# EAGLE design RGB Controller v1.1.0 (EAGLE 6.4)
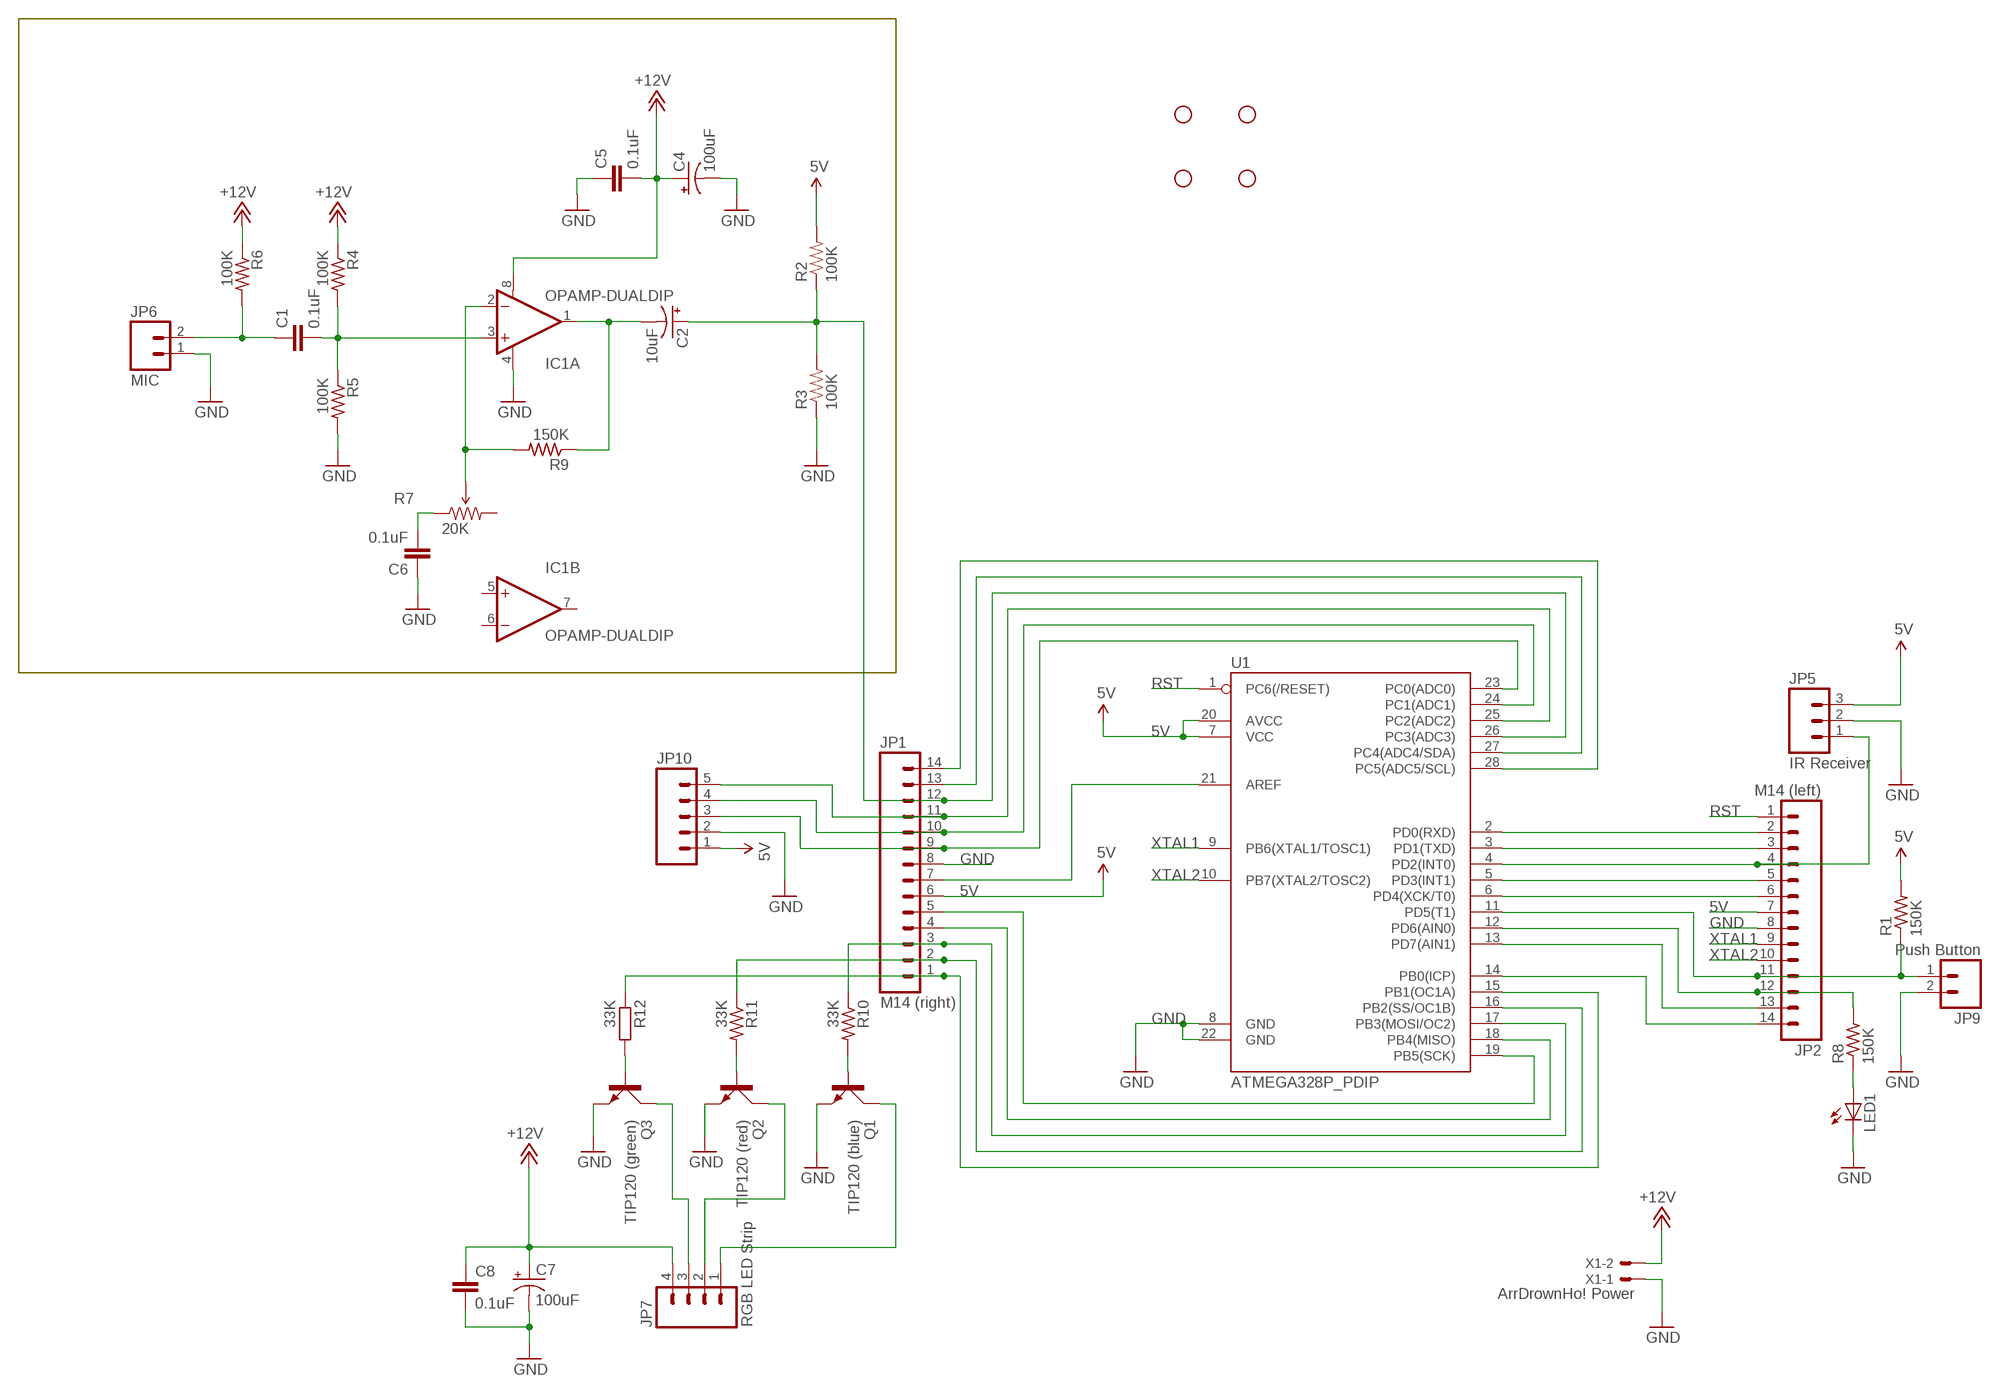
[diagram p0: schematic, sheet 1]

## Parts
C1  0.1uF  CAPPTH  [CAP-PTH-SMALL]
C2  10uF  CAP_POLPTH2  [CPOL-RADIAL-10UF-25V]
C4  100uF  CAP_POLPTH1  [CPOL-RADIAL-100UF-25V]
C5  0.1uF  CAPPTH  [CAP-PTH-SMALL]
C6  0.1uF  CAPPTH  [CAP-PTH-SMALL]
C7  100uF  CAP_POLPTH1  [CPOL-RADIAL-100UF-25V]
C8  0.1uF  CAPPTH  [CAP-PTH-SMALL]
IC1  OPAMP-DUALDIP  [DIP08]
JP1  M14 (right)  M14  [1X14]
JP2  M14 (left)  M14  [1X14]
JP5  IR Receiver  M03PTH  [1X03]
JP6  MIC  M02PTH  [1X02]
JP7  RGB LED Strip  M04PTH  [1X04]
JP9  Push Button  M02PTH  [1X02]
JP10  M05PTH  [1X05]
LED1  LED3MM  [LED3MM]
Q1  TIP120 (blue)  TIP41C  [TO220AV]
Q2  TIP120 (red)  TIP41C  [TO220AV]
Q3  TIP120 (green)  TIP41C  [TO220AV]
R1  150K  R-US_0207/2V  [0207/2V]
R2  100K  RESISTORAXIAL-0.3  [AXIAL-0.3]
R3  100K  RESISTORAXIAL-0.3  [AXIAL-0.3]
R4  100K  R-US_0207/2V  [0207/2V]
R5  100K  R-US_0207/2V  [0207/2V]
R6  100K  R-US_0207/2V  [0207/2V]
R7  20K  TRIMPOTPTH  [TRIM_POT_PTH]
R8  150K  R-US_0207/2V  [0207/2V]
R9  150K  R-US_0207/2V  [0207/2V]
R10  33K  R-US_0207/2V  [0207/2V]
R11  33K  R-US_0207/2V  [0207/2V]
R12  33K  R-EU_0411/3V  [0411V]
STANDOFF1  STAND-OFF  [STAND-OFF]
STANDOFF2  STAND-OFF  [STAND-OFF]
STANDOFF3  STAND-OFF  [STAND-OFF]
STANDOFF4  STAND-OFF  [STAND-OFF]
U1  ATMEGA328P_PDIP  [DIL28-3]
X1  ArrDrownHo! Power  C-GRID-02-70543  [70543-02]

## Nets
5V: JP1.6 JP2.7 JP5.3 JP10.1 R1.2 R2.P$2 U1.7(VCC) U1.20(AVCC)
+12V: C4.1(+) C5.2 C7.1(+) C8.1 IC1.8(A:V+) JP7.4 R4.1 R6.1 X1.2
AREF: JP1.7 U1.21(AREF)
GND: C4.2(-) C5.1 C6.1 C7.2(-) C8.2 IC1.4(A:V-) JP1.8 JP2.8 JP5.2 JP6.1 JP9.2 JP10.2 LED1.K(C) Q1.E Q2.E Q3.E R3.P$1 R5.2 U1.8(GND) U1.22(GND) X1.1
N$1: JP2.2 U1.2(PD0(RXD))
N$2: JP2.3 U1.3(PD1(TXD))
N$3: JP2.4 JP5.1 U1.4(PD2(INT0))
N$4: JP2.5 U1.5(PD3(INT1))
N$5: JP2.6 U1.6(PD4(XCK/T0))
N$6: LED1.A R8.1
N$7: JP2.12 R8.2 U1.12(PD6(AIN0))
N$8: JP2.13 U1.13(PD7(AIN1))
N$9: JP1.9 JP10.3 U1.23(PC0(ADC0))
N$10: JP1.10 JP10.4 U1.24(PC1(ADC1))
N$11: JP1.11 JP10.5 U1.25(PC2(ADC2))
N$12: JP7.2 Q2.C
N$13: JP1.13 U1.27(PC4(ADC4/SDA))
N$14: JP1.14 U1.28(PC5(ADC5/SCL))
N$15: JP1.1 R12.1 U1.15(PB1(OC1A))
N$16: JP2.14 U1.14(PB0(ICP))
N$17: JP1.5 U1.19(PB5(SCK))
N$18: JP1.4 U1.18(PB4(MISO))
N$19: JP1.3 R10.1 U1.17(PB3(MOSI/OC2))
N$20: JP1.2 R11.1 U1.16(PB2(SS/OC1B))
N$21: C2.1(+) JP1.12 R2.P$1 R3.P$2 U1.26(PC3(ADC3))
N$22: C2.2(-) IC1.1(A:OUT) R9.1
N$25: IC1.2(A:-IN) R7.2(WIPER) R9.2
N$26: Q2.B R11.2
N$27: C1.2 IC1.3(A:+IN) R4.2 R5.1
N$28: C1.1 JP6.2 R6.2
N$29: C6.2 R7.1(CCW)
N$30: Q3.B R12.2
N$31: Q1.B R10.2
N$33: JP7.3 Q3.C
N$35: JP7.1 Q1.C
N$37: JP2.11 JP9.1 R1.1 U1.11(PD5(T1))
RST: JP2.1 U1.1(PC6(/RESET))
XTAL1: JP2.9 U1.9(PB6(XTAL1/TOSC1))
XTAL2: JP2.10 U1.10(PB7(XTAL2/TOSC2))
Unconnected: IC1.5(B:+IN) IC1.6(B:-IN) IC1.7(B:OUT) R7.3(CW)

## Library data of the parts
C1 C5 C6 C8 = SparkFun-Capacitors:CAP: Capacitor
C2 C4 C7 = SparkFun-Capacitors:CAP_POL: Capacitor Polarized
IC1 = SparkFun-AnalogIC:OPAMP-DUAL: Generic op-amp footprint
JP1 JP2 = SparkFun-Connectors:M14: Header 14 Standard 14-pin 0.1" header. Use with straight break away headers (SKU : PRT-00116), right angle break away headers (PRT-00553), swiss pins (PRT-00743), machine pins (PRT-00117), and female headers (PRT-00115).
JP5 = SparkFun-Connectors:M03: Header 3 Standard 3-pin 0.1" header. Use with straight break away headers (SKU : PRT-00116), right angle break away headers (PRT-00553), swiss pins (PRT-00743), machine pins (PRT-00117), and female headers (PRT-00115). Molex polarized connector foot print use with SKU : PRT-08232 with associated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
JP6 JP9 = SparkFun-Connectors:M02: Header 2
JP7 = SparkFun-Connectors:M04: Header 4 Standard 4-pin 0.1" header. Use with straight break away headers (SKU : PRT-00116), right angle break away headers (PRT-00553), swiss pins (PRT-00743), machine pins (PRT-00117), and female headers (PRT-00115). Molex polarized connector foot print use with SKU : PRT-08231 with associated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
JP10 = SparkFun-Connectors:M05: Header 5 Standard 5-pin 0.1" header. Use with straight break away headers (SKU : PRT-00116), right angle break away headers (PRT-00553), swiss pins (PRT-00743), machine pins (PRT-00117), and female headers (PRT-00115). Molex polarized connector foot print use with SKU : PRT-08230 with associated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
LED1 = SparkFun-LED:LED: LEDs
Q1-Q3 = transistor-power:TIP41C: NPN TRANSISTOR
R1 R4-R6 R8-R11 = resistor:R-US_: RESISTOR, American symbol
R2 R3 = SparkFun-Passives:RESISTOR: Resistor
R7 = SparkFun-Electromechanical:TRIMPOT: Various small potentiometers for "set-and-forget" applications
R12 = resistor:R-EU_: RESISTOR, European symbol
STANDOFF1-STANDOFF4 = SparkFun-Electromechanical:STAND-OFF: #4 Stand Off
U1 = SparkFun-DigitalIC:ATMEGA328P_PDIP: uC used in the Arduino 32kb flash, 1k EEPROM, 2k SRAM This is the through-hole version of this chip.
X1 = con-molex:C-GRID-02: CONNECTOR; OC_FARNELL: unknown; OC_NEWARK: unknown

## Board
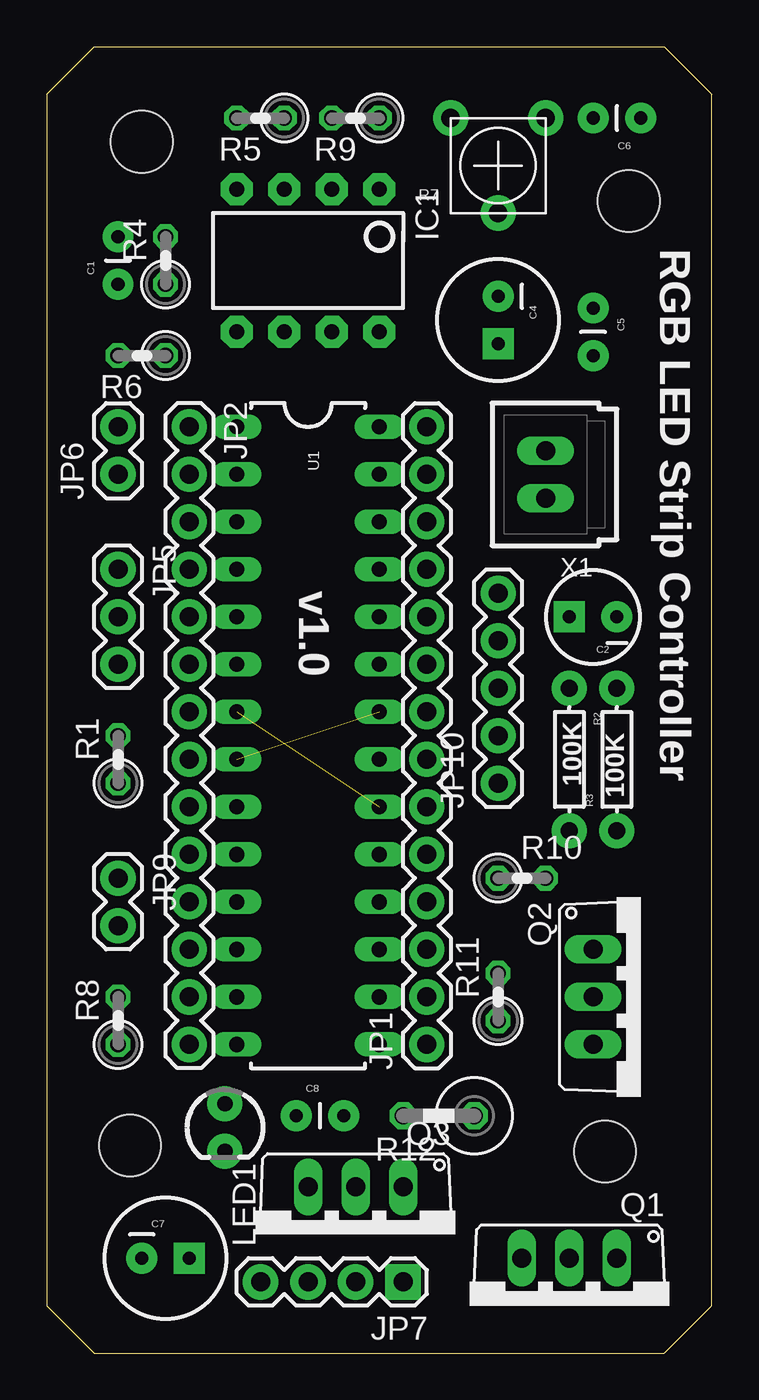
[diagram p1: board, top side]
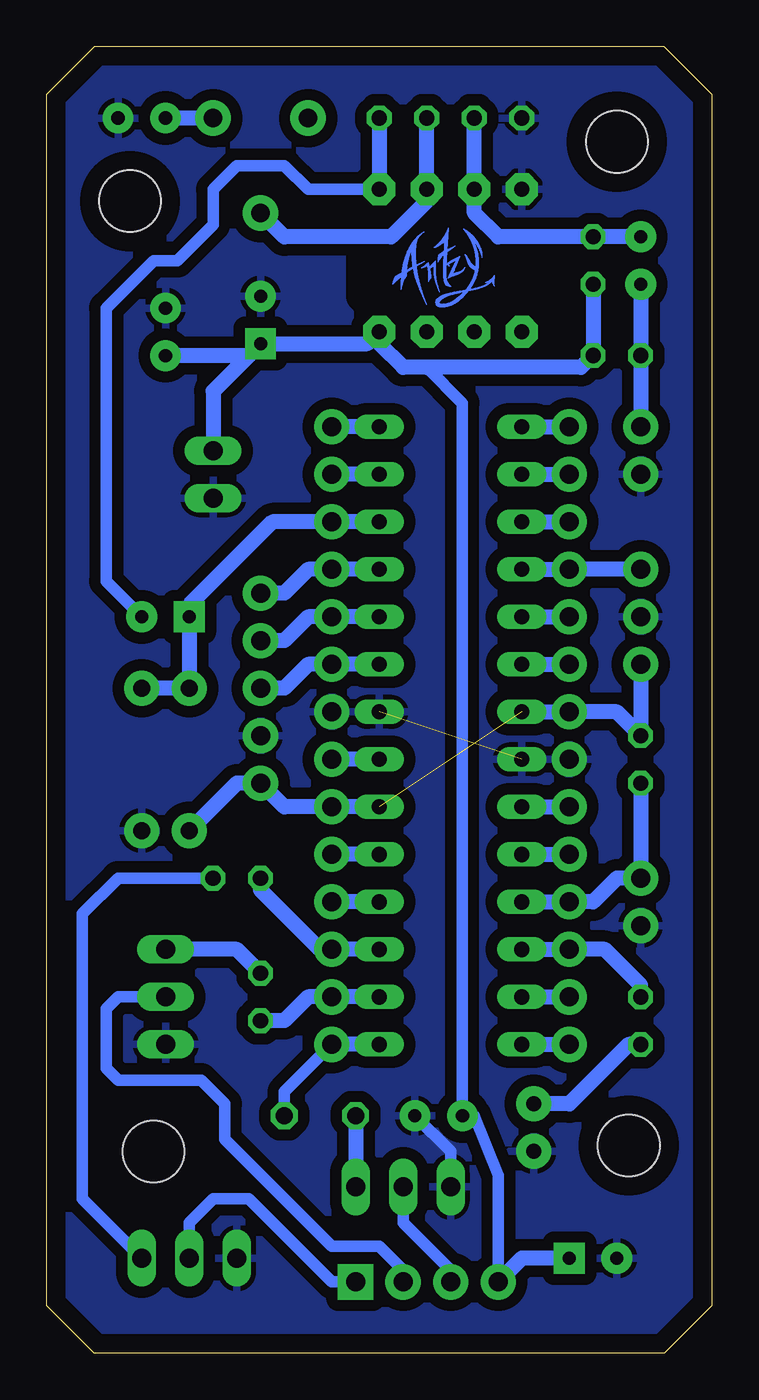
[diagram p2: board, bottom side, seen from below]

Size 35.56 x 69.85 mm. Coordinates in mm from the lower left corner, seen from the top.
Outline: 35.56,2.54 35.56,67.31 33.02,69.85 2.54,69.85 0,67.31 0,2.54 2.54,0 33.02,0 35.56,2.54
Copper layers (1*16): Top 0.035mm / dielectric 1.5mm / Bottom 0.035mm
Design rules "default *": minimum track width 10mil, minimum drill 24mil, track to track 8mil, track to pad 8mil, pad to pad 8mil, via to via 8mil, smd to smd 8mil, copper to edge 40mil, drill to drill 8mil, minimum pad ring 10mil, minimum via ring 8mil, stop-mask expansion 4mil, vias tented up to drill 0mil, thermal gap 10mil
bRestrict: area 17.5,56.1 to 18.9,58.7

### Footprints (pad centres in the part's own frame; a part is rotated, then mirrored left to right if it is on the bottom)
CAP-PTH-SMALL = drill 0.7 pad 1.651: 1 0,0; 2 2.54,0
CPOL-RADIAL-10UF-25V = drill 0.7 pad 1.651 square: 1 1.27,0 | drill 0.7 pad 1.651: 2 -1.27,0
CPOL-RADIAL-100UF-25V = drill 0.7 pad 1.651 square: 1 1.27,0 | drill 0.7 pad 1.651: 2 -1.27,0
DIP08 = drill 0.813 pad 1.727 octagon: 1 -3.81,-3.81; 2 -1.27,-3.81; 3 1.27,-3.81; 4 3.81,-3.81; 5 3.81,3.81; 6 1.27,3.81; 7 -1.27,3.81; 8 -3.81,3.81
1X14 = drill 1.016 pad 1.88: 1 0,0; 2 2.54,0; 3 5.08,0; 4 7.62,0; 5 10.16,0; 6 12.7,0; 7 15.24,0; 8 17.78,0; 9 20.32,0; 10 22.86,0; 11 25.4,0; 12 27.94,0; 13 30.48,0; 14 33.02,0
1X03 = drill 1.016 pad 1.88: 1 0,0; 2 2.54,0; 3 5.08,0
1X02 = drill 1.016 pad 1.88: 1 0,0; 2 2.54,0
1X04 = drill 1.016 pad 1.88 square: 1 0,0 | drill 1.016 pad 1.88: 2 2.54,0; 3 5.08,0; 4 7.62,0
1X05 = drill 1.016 pad 1.88: 1 0,0; 2 2.54,0; 3 5.08,0; 4 7.62,0; 5 10.16,0
LED3MM = drill 0.813 pad 1.88: A -1.27,0; K 1.27,0
TO220AV = drill 1.016 long: B -2.54,-2.54; C 0,-2.54; E 2.54,-2.54
0207/2V = drill 0.813 octagon: 1 -1.27,0; 2 1.27,0
AXIAL-0.3 = drill 0.9 pad 1.88: P$1 -3.81,0; P$2 3.81,0
TRIM_POT_PTH = drill 1 pad 1.88: 1 -2.54,-2.54; 2 0,2.54; 3 2.54,-2.54
0411V = drill 0.914 octagon: 1 -2.54,0; 2 1.27,0
STAND-OFF = hole 3.302: 0,0
DIL28-3 = drill 0.813 long: 1 -16.51,-3.81; 2 -13.97,-3.81; 3 -11.43,-3.81; 4 -8.89,-3.81; 5 -6.35,-3.81; 6 -3.81,-3.81; 7 -1.27,-3.81; 8 1.27,-3.81; 9 3.81,-3.81; 10 6.35,-3.81; 11 8.89,-3.81; 12 11.43,-3.81; 13 13.97,-3.81; 14 16.51,-3.81; 15 16.51,3.81; 16 13.97,3.81; 17 11.43,3.81; 18 8.89,3.81; 19 6.35,3.81; 20 3.81,3.81; 21 1.27,3.81; 22 -1.27,3.81; 23 -3.81,3.81; 24 -6.35,3.81; 25 -8.89,3.81; 26 -11.43,3.81; 27 -13.97,3.81; 28 -16.51,3.81
70543-02 = drill 1.016 long: 1 -1.27,0; 2 1.27,0

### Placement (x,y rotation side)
C1  3.81,57.15 90 top
C2  29.21,39.37 180 top
C4  24.13,55.24 270 top
C5  29.21,55.88 270 top
C6  31.75,66.04 180 top
C7  6.35,5.08 0 top
C8  13.34,12.7 0 top
IC1  13.97,58.42 180 top
JP1  20.32,16.51 90 top
JP2  7.62,49.53 270 top
JP5  3.81,41.91 270 top
JP6  3.81,46.99 90 top
JP7  19.05,3.81 180 top
JP9  3.81,25.4 270 top
JP10  24.13,30.48 90 top
LED1  9.53,12.06 270 top
Q1  27.94,2.54 180 top
Q2  31.75,19.05 270 top
Q3  16.51,6.35 180 top
R1  3.81,31.75 90 top
R2  27.94,31.75 270 top
R3  30.48,31.75 90 top
R4  6.35,58.42 90 top
R5  11.43,66.04 180 top
R6  5.08,53.34 180 top
R7  24.13,63.5 180 top
R8  3.81,17.78 90 top
R9  16.51,66.04 180 top
R10  25.4,25.4 0 top
R11  24.13,19.05 90 top
R12  20.32,12.7 180 top
STANDOFF1  4.45,11.11 0 top
STANDOFF2  29.84,10.79 0 top
STANDOFF3  5.08,64.77 0 top
STANDOFF4  31.11,61.59 0 top
U1  13.97,33.02 270 top
X1  26.67,46.99 90 top

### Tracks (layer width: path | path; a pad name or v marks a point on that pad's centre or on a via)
5V  (1 unrouted)
  Bottom 0.813: U1.20 JP1.6 22.86,29.21 JP10.1 25.4,30.48 R2.P$2 | U1.7 JP2.7 5.08,34.29 R1.2 JP5.3
+12V
  Bottom 0.61: 15.24,52.7 13.34,50.8 C8.1 12.7,12.7 11.43,9.53 JP7.4
  Bottom 0.813: R4.1 R6.1 6.99,52.7 15.24,52.7 16.51,52.7 17.78,53.98 IC1.8 18.41,53.98 C4.1 24.77,53.34 | 24.77,53.34 C5.2 | 24.77,53.34 26.67,51.44 X1.2 | C7.1 10.16,5.08 JP7.4
AREF
  Bottom 0.813: U1.21 JP1.7
GND  (1 unrouted)
  Bottom 0.61: Q3.E 13.97,10.79 C8.2
  pour Bottom (isolate 0.61): 33.02,0 35.56,2.54 35.56,67.31 33.02,69.85 2.54,69.85 0,67.31 0,2.54 2.54,0
N$1
  Bottom 0.813: U1.2 JP2.2
N$2
  Bottom 0.813: U1.3 JP2.3
N$3
  Bottom 0.813: U1.4 JP2.4 JP5.1
N$4
  Bottom 0.813: U1.5 JP2.5
N$5
  Bottom 0.813: U1.6 JP2.6
N$6
  Bottom 0.813: R8.1 4.45,16.51 7.62,13.34 LED1.A
N$7
  Bottom 0.813: U1.12 JP2.12 5.71,21.59 3.81,19.68 R8.2
N$8
  Bottom 0.813: U1.13 JP2.13
N$9
  Bottom 0.813: U1.23 JP1.9 21.59,36.83 22.86,35.56 JP10.3
N$10
  Bottom 0.813: U1.24 JP1.10 21.59,39.37 22.86,38.1 JP10.4
N$11
  Bottom 0.813: U1.25 JP1.11 21.59,41.91 22.86,40.64 JP10.5
N$12
  Bottom 0.61: JP7.2 16.51,4.45 17.78,5.71 20.32,5.71 26.04,11.43 26.04,13.34 27.3,14.61 31.75,14.61 32.38,15.24 32.38,18.41 31.75,19.05 Q2.C
N$13
  Bottom 0.813: U1.27 JP1.13
N$14
  Bottom 0.813: U1.28 JP1.14
N$15
  Bottom 0.61: JP1.1 22.86,13.97 R12.1
  Bottom 0.813: U1.15 JP1.1
N$16
  Bottom 0.813: U1.14 JP2.14
N$17
  Bottom 0.813: U1.19 JP1.5
N$18
  Bottom 0.813: U1.18 JP1.4
N$19
  Bottom 0.813: U1.17 JP1.3 20.95,21.59 24.13,24.77 R10.1
N$20
  Bottom 0.813: U1.16 JP1.2 21.59,19.05 22.86,17.78 R11.1
N$21
  Bottom 0.813: U1.26 JP1.12 23.5,44.45 27.94,40.01 C2.1 R2.P$1 R3.P$2
N$22
  Bottom 0.61: IC1.1 21.59,62.23 22.86,63.5 25.4,63.5 26.67,62.23 26.67,60.33 28.57,58.42 29.84,58.42 32.38,55.88 32.38,41.27 C2.2
  Bottom 0.813: R9.1 IC1.1
N$25
  Bottom 0.813: R9.2 IC1.2 15.24,61.59 17.14,59.69 22.86,59.69 R7.2
N$26
  Bottom 0.813: R11.2 25.4,21.59 Q2.B
N$27
  Bottom 0.813: C1.2 R4.2 11.43,59.69 12.7,60.96 IC1.3 R5.1
N$28
  Bottom 0.813: C1.1 R6.2 JP6.2
N$29
  Bottom 0.813: R7.1 C6.2
N$30
  Bottom 0.813: R12.2 Q3.B
N$31
  Bottom 0.61: R10.2 31.75,25.4 33.66,23.5 33.66,8.26 Q1.B
N$33
  Bottom 0.61: Q3.C 16.51,6.99 13.97,4.45 JP7.3
N$35
  Bottom 0.61: JP7.1 20.32,3.81 24.77,8.26 26.67,8.26 27.94,6.99 Q1.C
N$37
  Bottom 0.813: U1.11 JP2.11 6.35,24.13 5.08,25.4 JP9.1 R1.1
RST
  Bottom 0.813: U1.1 JP2.1
XTAL1
  Bottom 0.813: U1.9 JP2.9
XTAL2
  Bottom 0.813: U1.10 JP2.10
(copper drawn outside any net)
  shapes: Bottom area x3066

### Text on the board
tPlace: RGB LED Strip Controller | v1.0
